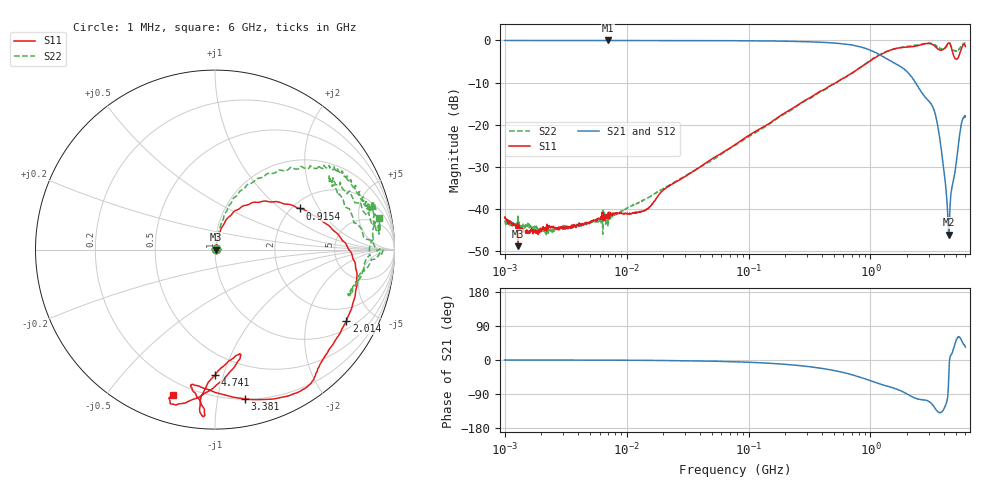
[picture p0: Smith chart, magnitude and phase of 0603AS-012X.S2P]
!s-Parameter Generated by FASTRON Sdn. Bhd.
!FASTRON P/N : 0603AS-012J
!s-Parameter Generated by FASTRON Sdn. Bhd.
!FASTRON P/N : 0603AS-012X
!Keysight Technologies: E5071C_MY46733604_B.14.02
!Date: Thu Nov 23 09:57:15 2023
!Version  :Rev01  Thu Nov 23 09:57:15 2023
!Data & Calibration Information:
!Freq  S11:SOLT2(ON)  S21:SOLT2(ON)  S12:SOLT2(ON)  S22:SOLT2(ON)
!PortZ  Port1:50+j0  Port2:50+j0
!When reading reference impedance value at option line is always used.
! Remarks : This data is being provided solely for informational purposes.
# Hz S dB R 50
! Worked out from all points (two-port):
!   1601 points, 1 MHz to 6 GHz, reference 50 ohm
!   highest |S21| = -0.04 dB at 7.017 MHz (marker M1); lowest = -46.0 dB at 4.377 GHz (marker M2)
!   |S21| within 3 dB of the highest: start of sweep to 1.123 GHz
!   lowest |S11| = -48.8 dB at 1.288 MHz (marker M3), VSWR 1.01, Z = 50.4 + j0.0257 ohm
!   |S11| at or under -10 dB: start of sweep to 523.8 MHz
!   |S22| runs from -46.0 to -0.6 dB; largest |S21 - S12| = 0.0073
!   S11 on the Smith chart (normalised r, x): 1 MHz: 1.02, +0.00; 915.4 MHz: 2.18, +1.38; 2.014 GHz: 1.32, -3.45; 3.381 GHz: 0.20, -1.20; 4.741 GHz: 0.34, -0.94; 6 GHz: 0.13, -0.74
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1000000  -41.98 17.1  -0.05 -0.0  -0.06 -0.1  -42.70 15.4
1287650  -48.76 4.0  -0.06 -0.1  -0.04 -0.0  -41.30 5.7
2190642  -44.47 25.6  -0.06 -0.2  -0.05 -0.2  -45.13 31.9
4277066  -43.94 34.7  -0.06 -0.3  -0.05 -0.3  -43.77 34.4
7017068  -40.91 52.4  -0.04 -0.5  -0.06 -0.6  -44.10 41.4
1.383558e7  -40.43 64.2  -0.06 -0.9  -0.07 -0.9  -37.82 52.7
1.823719e7  -36.75 65.4  -0.06 -1.2  -0.07 -1.1  -35.78 62.4
7.757876e7  -24.73 75.7  -0.11 -4.6  -0.11 -4.6  -24.87 76.7
3.307917e8  -13.33 64.8  -0.37 -18.5  -0.37 -18.4  -13.54 74.2
5.990366e8  -9.01 47.9  -0.85 -33.0  -0.85 -33.0  -9.02 67.0
9.153647e8  -5.62 26.0  -1.93 -50.5  -1.93 -50.5  -5.53 53.2
1.414819e9  -2.45 -0.7  -4.67 -70.5  -4.68 -70.5  -2.46 36.9
2.013714e9  -1.58 -28.6  -7.60 -90.5  -7.60 -90.4  -1.41 26.6
2.951149e9  -0.71 -56.4  -14.11 -108.1  -14.08 -108.0  -0.83 14.9
3.381472e9  -1.44 -78.7  -17.31 -127.0  -17.30 -127.1  -1.04 3.8
3.867453e9  -2.32 -99.9  -27.39 -135.8  -27.40 -135.9  -2.00 -17.8
4.252188e9  -1.03 -93.9  -38.90 -105.5  -38.94 -105.7  -1.21 -4.5
4.377169e9  -0.63 -93.8  -46.00 -48.0  -46.03 -47.8  -0.69 -0.9
4.740907e9  -3.10 -90.1  -33.76 24.7  -33.79 24.6  -2.13 16.9
5.244544e9  -4.08 -77.2  -24.96 61.7  -24.97 61.8  -2.30 31.4
5.608282e9  -1.72 -95.6  -19.40 50.7  -19.41 50.9  -1.10 13.6
6e9  -1.49 -106.1  -18.17 34.3  -18.16 34.4  -0.63 10.7
